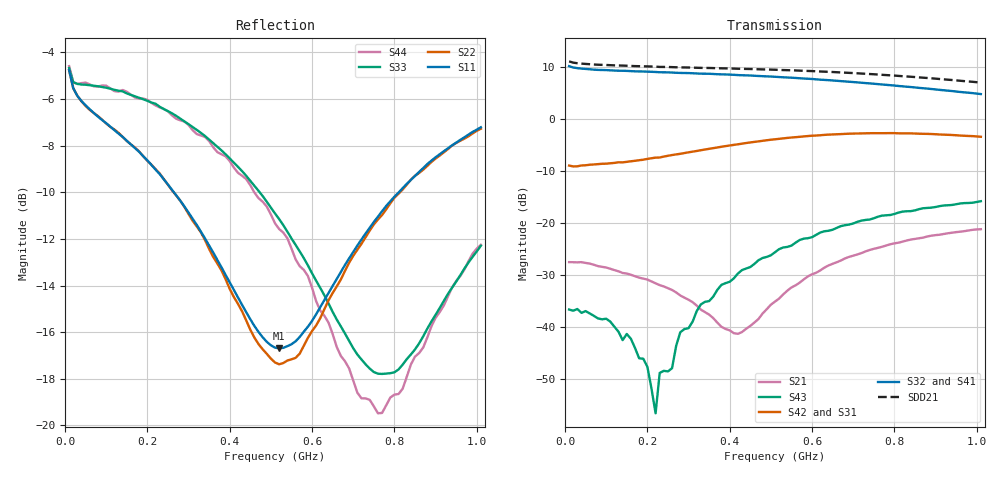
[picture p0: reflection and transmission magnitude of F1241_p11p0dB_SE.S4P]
! Integrated Device Technology
! Corporate Headquarters
! 6024 Silver Creek Valley Road
! San Jose, CA 95138  USA
! Phone:  1-408-284-8200
! Toll Free:  1-800-223-1366
! Webpage:  http://www.idt.com/
! Timing and RF Division
! 515 Groton Road, Suite 102
! Westford, MA 01886-6024
! Device:  F1241
! Description: Dual Intermediate Frequency Digital Variable Gain Amplifier
! Frequency:  10.0 -  500.00 MHz
! Package:  5x5 mm QFN Plastic Package: 32 pin
! Ports:  8 RF, 20 DC
!  Pin  1  = GA3  Pin 17  = RF OUT_B+
!  Pin  2  = GA4  Pin 18  = RF OUT_B-
!  Pin  3  = GA5  Pin 19  = STBY_B
!  Pin  4  = ISET_A  Pin 20  = Ground
!  Pin  5  = ISET_B  Pin 21  = Ground
!  Pin  6  = GB5  Pin 22  = STB_A
!  Pin  7  = GB4  Pin 23  = RF OUT_A-  = Port 4
!  Pin  8  = GB3  Pin 24  = RF OUT_A+  = Port 3
!  Pin  9  = GB2  Pin 25  = NO CONNECT
!  Pin 10  = GB1  Pin 26  = NO CONNECT
!  Pin 11  = RF IN_B+  Pin 27  = VCC
!  Pin 12  = RF IN_B-  Pin 28  = Ground
!  Pin 13  = Ground  Pin 29  = RF IN_A-  = Port 2
!  Pin 14  = VCC  Pin 30  = RF IN_A+  = Port 1
!  Pin 15  = NO CONNECT  Pin 31  = GA1
!  Pin 16  = NO CONNECT  Pin 32  = GA2
! State:  9
! Gain State:  11.0 dB
! Voltages:  Vcc = +5.00 Volts  Icc approximately 160.0 mA or 80 mA per channel.
! Data:  The device was measured on a custom evaluation board which has
!  individual transmission lines to the RF pins.  Data was collected
!  using a calibrated network analyzer.  The evaluation board was
!  de-embedded using a port reference technique.
!  The reference plane is the edge of the package pin.
!  Only Channel A was measured.
!  This data is in single-ended operation.  If your needs are balanced
!  or differential S-parameters then this file needs to be used a
!  linear simulator.
! Misc:  Lot Code  160028MY
!  Action Tracker AT004
! Date Measured:  2014-08-14
! Date:  2014-08-28  MJV
! Note:
!  Integrated Device Technology supplies this data as a sample of measured
!  data at the package pin for this product.  Your particular data for this
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# Hz S dB R 50
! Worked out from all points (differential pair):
!   101 points, 10 MHz to 1.01 GHz, reference 50 ohm
!   strongest paths, dB at 10 MHz, 260 MHz, 510 MHz, 760 MHz, 1.01 GHz:
!     S32: 10.2, 8.9, 8.1, 6.7, 4.8
!     S41: 10.2, 8.9, 8.0, 6.6, 4.6
!     S42: -9.0, -6.9, -3.9, -2.7, -3.4
!     S31: -9.0, -7.0, -4.1, -2.9, -3.6
!     S43: -36.7, -48.0, -25.6, -18.8, -15.8
!     S21: -27.6, -32.9, -35.1, -24.8, -21.2
!   taken as a pair (ports 2,1 in; 3,4 out), SDD21 dB: 11.1, 10.0, 9.5, 8.5, 7.0
!   lowest |S11| = -16.7 dB at 520 MHz (marker M1), VSWR 1.34, Z = 39.8 - j8.42 ohm
!   |S11| at or under -10 dB: 264.4 MHz to 810.8 MHz (546.4 MHz wide, 102 % of centre)
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1e7  -4.76 -17.1  -27.58 5.0  -50.58 46.5  -19.18 11.5
     -27.55 4.9  -4.77 -17.0  -19.20 11.2  -50.73 45.6
     -8.98 1.2  10.16 -178.8  -4.67 -14.8  -36.61 37.1
     10.18 -178.7  -8.97 1.3  -36.67 36.1  -4.59 -14.9
1.9e8  -8.46 -36.8  -30.73 -18.2  -34.62 58.7  -19.62 -9.3
       -30.72 -20.4  -8.46 -35.4  -19.57 -9.2  -34.66 58.6
       -7.89 2.2  9.13 151.9  -6.01 -18.7  -45.59 -22.4
       9.09 151.3  -7.85 2.0  -46.13 12.2  -5.98 -17.8
2.3e8  -9.22 -43.4  -31.92 -17.8  -33.10 55.6  -19.55 -11.0
       -31.98 -22.0  -9.20 -41.5  -19.52 -10.9  -33.15 54.9
       -7.50 1.5  8.99 146.5  -6.34 -22.7  -53.44 4.7
       8.96 145.9  -7.42 1.2  -48.86 72.1  -6.37 -21.5
2.4e8  -9.45 -45.2  -32.17 -17.7  -32.78 55.1  -19.53 -11.2
       -32.23 -22.4  -9.44 -43.2  -19.49 -11.3  -32.81 54.4
       -7.32 1.2  8.98 145.2  -6.43 -23.5  -80.80 7.5
       8.94 144.6  -7.24 0.9  -48.46 83.6  -6.43 -22.3
3e8  -10.87 -56.6  -34.32 -15.2  -31.04 50.0  -19.35 -13.6
     -34.78 -21.5  -10.93 -54.2  -19.31 -13.8  -31.05 49.0
     -6.53 -1.3  8.83 137.4  -7.08 -29.3  -42.29 142.5
     8.77 136.7  -6.42 -1.9  -40.25 121.1  -7.12 -28.5
5.2e8  -16.69 -135.1  -33.50 65.7  -27.12 28.6  -18.70 -27.8
       -34.56 77.9  -17.38 -133.0  -18.53 -27.7  -27.04 26.7
       -3.98 -20.8  8.06 108.4  -11.15 -56.2  -26.57 117.9
       7.96 107.6  -3.83 -22.5  -25.05 109.4  -11.58 -53.2
1.01e9  -7.21 119.0  -21.72 44.2  -24.13 -13.4  -19.53 -66.0
        -21.21 46.2  -7.28 118.4  -19.03 -66.6  -24.09 -17.7
        -3.57 -83.6  4.79 49.8  -12.29 157.2  -16.55 52.9
        4.59 49.1  -3.43 -87.0  -15.83 48.2  -12.25 150.7
